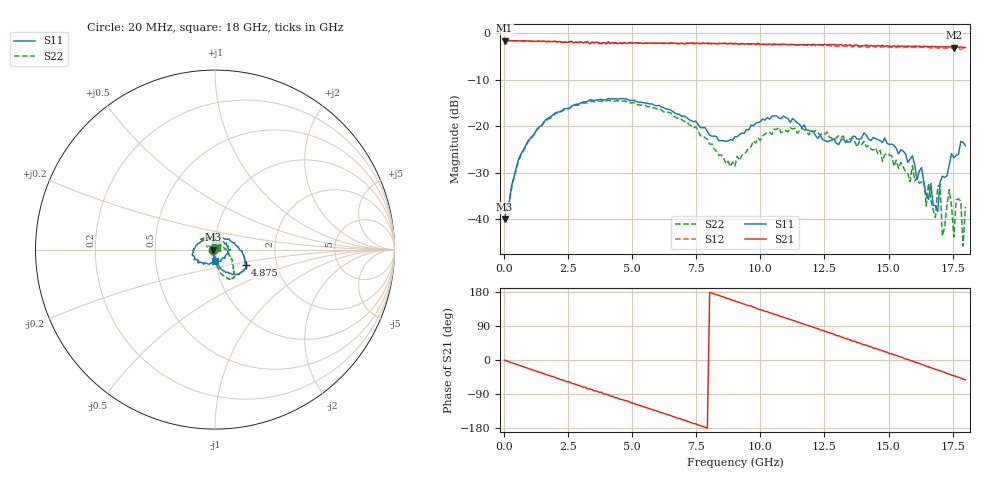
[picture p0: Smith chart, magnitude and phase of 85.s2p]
!Agilent Technologies,N5230A,US43500223,A.07.50.48
!Agilent N5230A: A.07.50.48
!Date: Tuesday, February 02, 2016 12:46:07
!Correction: S11(Full 2 Port(1,2))
!S21(Full 2 Port(1,2))
!S12(Full 2 Port(1,2))
!S22(Full 2 Port(1,2))
!S2P File: Measurements: S11, S21, S12, S22:
# Hz S  RI  R 50
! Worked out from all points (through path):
!   201 points, 20 MHz to 18 GHz, reference 50 ohm
!   highest |S21| = -1.54 dB at 20 MHz (marker M1); lowest = -3.1 dB at 17.55 GHz (marker M2)
!   group delay of S21, straight-line fit = 63.3 ps
!   lowest |S11| = -40.0 dB at 20 MHz (marker M3), VSWR 1.02, Z = 49 + j0.0122 ohm
!   |S11| at or under -10 dB: start of sweep to end of sweep
!   |S22| runs from -45.8 to -14.4 dB; largest |S21 - S12| = 0.075
!   S11 on the Smith chart (normalised r, x): 20 MHz: 0.98, +0.00; 4.875 GHz: 1.38, -0.25; 18 GHz: 0.99, -0.12
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2e7  -0.01 0.000124  0.8374 -0.00674  0.8387 -0.0105  -0.0114 -0.000359
9.19e8  0.00996 -0.068  0.7715 -0.3066  0.7678 -0.3111  0.000312 -0.0671
3.0766e9  0.1181 -0.1399  0.246 -0.7505  0.2425 -0.7616  0.0739 -0.1617
4.8746e9  0.1703 -0.0866  -0.2686 -0.7512  -0.2831 -0.7296  0.1056 -0.1484
6.0433e9  0.1646 -0.0362  -0.5711 -0.5383  -0.5844 -0.5208  0.109 -0.1107
9.01e9  -0.0418 0.0653  -0.7144 0.3183  -0.6891 0.3394  0.011 0.036
1.05383e10  -0.1263 -0.0295  -0.3933 0.6622  -0.3623 0.6573  -0.0697 0.0615
1.20666e10  -0.0324 -0.0817  0.0471 0.7617  0.0955 0.7431  -0.056 0.0675
1.50333e10  0.0495 0.0405  0.6948 0.2144  0.686 0.1646  -0.0151 0.047
1.63818e10  0.00354 0.0243  0.7055 -0.1674  0.6688 -0.2237  0.0137 0.022
1.64717e10  -0.00601 0.0174  0.697 -0.2006  0.6605 -0.2442  -0.000984 0.0139
1.65616e10  -0.0132 0.00973  0.6847 -0.2228  0.6481 -0.2723  0.00171 0.0244
1.68313e10  -0.0137 -0.00321  0.6563 -0.3051  0.6178 -0.3448  0.00811 0.00673
1.69212e10  -0.0116 -0.00377  0.64 -0.3215  0.5855 -0.3702  0.00447 0.0221
1.70111e10  -0.014 -0.0208  0.6332 -0.3394  0.5865 -0.3742  0.0187 0.0147
1.7101e10  -0.0154 -0.0247  0.6134 -0.3704  0.5622 -0.4091  0.00617 -0.00245
1.73707e10  -0.00191 -0.0389  0.5703 -0.4347  0.5076 -0.4673  0.0184 0.00989
1.75505e10  -0.00736 -0.0453  0.5258 -0.4652  0.4654 -0.4955  -0.00321 0.00561
1.77303e10  0.00252 -0.0501  0.4928 -0.507  0.4254 -0.5392  0.0149 -0.00738
1.78202e10  0.00694 -0.0685  0.4809 -0.5265  0.4072 -0.5326  0.0134 -0.00807
1.79101e10  7.94e-05 -0.0676  0.4488 -0.5462  0.3967 -0.567  0.0025 -0.00451
1.8e10  -0.000802 -0.062  0.432 -0.5535  0.3642 -0.5702  0.0117 0.00696
